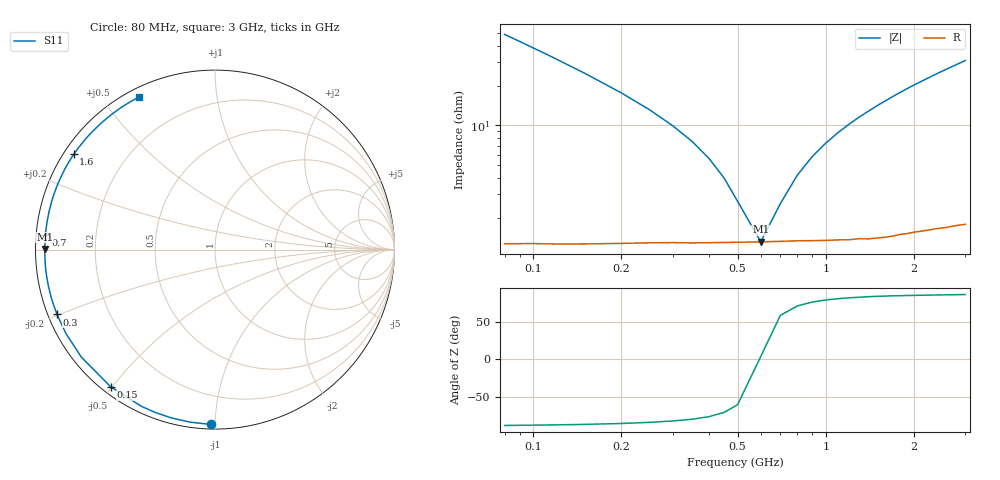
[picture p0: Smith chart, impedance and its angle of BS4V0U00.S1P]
! SIEMENS Small Signal Semiconductors
! BB640
! Si Tuning Diode in SOD323
! VR = 4 V
! S-Parameters:  July  1993
# GHz  S  MA  R  50
!  f  S11
! GHz  MAG  ANG
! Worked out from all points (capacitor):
!   33 points, 80 MHz to 3 GHz, reference 50 ohm
!   read as one part to ground: C = 40 pF near 80 MHz
!   lowest |Z| = 1.31 ohm at 600 MHz (marker M1)
!   series resonance near 596.4 MHz, so ESL is about 1.8 nH
!   S11 on the Smith chart (normalised r, x): 80 MHz: 0.03, -0.98; 150 MHz: 0.03, -0.50; 300 MHz: 0.03, -0.20; 700 MHz: 0.03, +0.04; 1.6 GHz: 0.03, +0.31; 3 GHz: 0.04, +0.62
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0.08  0.9744 -91.4
0.09  0.9714 -98.3
0.1  0.9687 -104.6
0.11  0.9666 -110.1
0.12  0.9647 -115.1
0.15  0.9603 -127.2
0.2  0.9557 -141.2
0.25  0.953 -150.7
0.3  0.9515 -157.7
0.35  0.951 -163.1
0.4  0.9503 -167.6
0.45  0.9498 -171.4
0.5  0.9495 -174.7
0.6  0.949 179.8
0.7  0.9487 175.0
0.8  0.9484 170.9
0.9  0.9486 167.1
1  0.9488 163.6
1.2  0.9492 157.2
1.4  0.9496 151.4
1.6  0.9494 146.0
1.8  0.9484 140.9
2  0.9481 136.2
2.2  0.9482 131.8
2.4  0.9483 127.6
2.6  0.9489 123.7
2.8  0.9491 120.0
3  0.9499 116.5
